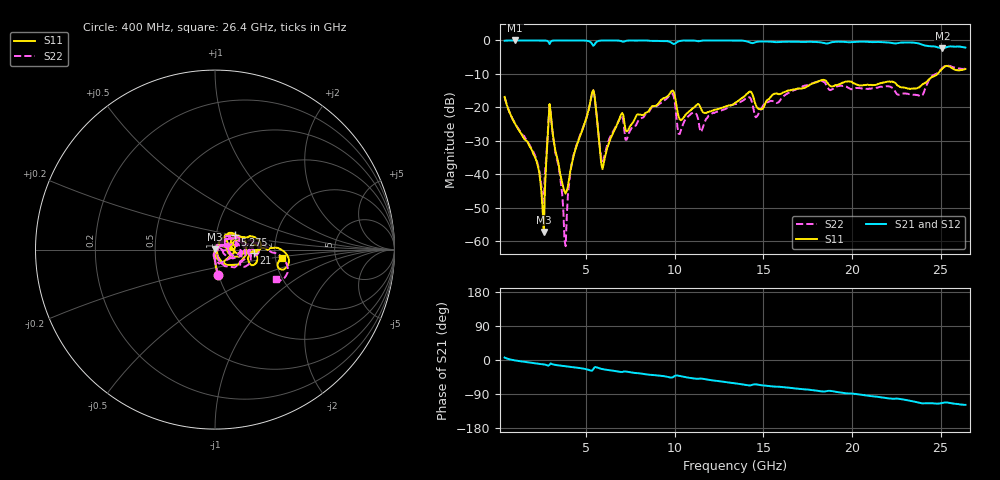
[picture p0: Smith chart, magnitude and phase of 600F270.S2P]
!  American Technical Ceramics  Date:  11/23/05
!  One Norden Lane
!  Huntington Station,  NY.  11746-2102
!  Tel:  (631) 622-4700  Fax:  (631) 622-4748
!  Part Number  600F270  Mounting Orientation: Horizontal
!  Description: Ultra Low ESR Microwave capacitors
!  Application: Coupling, Bypass, Tuning, DC Block
!  Filters, Matching
# GHZ S DB R 50
! Freq  |S11|  S11 Ph  |S21|  S21 Ph  |S12|  S12 Ph  |S22|  S22 Ph
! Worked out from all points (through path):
!   401 points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, 400 MHz to 26.4 GHz, reference 50 ohm
!   highest |S21| = 0.00 dB at 985 MHz (marker M1); lowest = -2.3 dB at 25.1 GHz (marker M2)
!   group delay of S21, straight-line fit = 12.9 ps
!   lowest |S11| = -57.1 dB at 2.61 GHz (marker M3), VSWR 1.00, Z = 50.1 + j0.0747 ohm
!   |S11| at or under -10 dB: start of sweep to 24.83 GHz
!   |S22| runs from -61.4 to -7.5 dB; largest |S21 - S12| = 0.0068
!   S11 on the Smith chart (normalised r, x): 400 MHz: 0.99, -0.29; 5.275 GHz: 1.23, +0.20; 21 GHz: 1.55, -0.06; 26.4 GHz: 2.16, -0.25
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0.4  -16.85 -83.4  -0.08 6.5  -0.08 6.5  -16.85 -83.2
0.985  -24.82 -91.1  0.00 -1.1  -0.01 -1.1  -24.72 -89.9
2.09  -34.56 -99.9  -0.01 -8.3  -0.01 -8.3  -34.05 -94.9
2.61  -57.15 32.5  -0.02 -11.6  -0.02 -11.7  -47.26 15.6
3  -21.52 -60.9  -0.39 -9.1  -0.41 -9.3  -21.74 -73.6
3.845  -45.71 -2.8  -0.01 -16.6  -0.01 -16.7  -61.40 60.2
4.235  -35.88 62.5  -0.01 -18.8  0.00 -18.8  -35.54 71.8
4.755  -27.19 62.3  -0.01 -22.1  -0.03 -22.1  -27.01 56.7
5.275  -17.28 35.8  -0.61 -28.2  -0.62 -28.1  -17.36 26.6
5.99  -36.68 20.9  -0.01 -24.7  -0.01 -24.7  -35.45 5.7
6.965  -22.18 46.6  -0.18 -31.5  -0.18 -31.5  -22.78 22.8
7.355  -26.88 42.7  -0.04 -31.3  -0.04 -31.3  -28.58 36.0
9.11  -18.58 50.6  -0.17 -41.5  -0.17 -41.5  -19.05 42.3
9.825  -15.10 16.8  -0.70 -46.3  -0.69 -46.2  -15.73 9.9
10.28  -23.54 -3.2  -0.18 -42.3  -0.18 -42.4  -27.93 15.9
13.4  -18.66 23.4  -0.01 -61.2  -0.01 -61.4  -18.99 27.6
17.755  -12.87 18.2  -0.43 -79.6  -0.44 -79.8  -12.80 9.9
21.005  -13.32 -4.6  -0.47 -95.0  -0.43 -95.2  -14.33 -4.4
22.11  -12.25 -14.2  -0.67 -101.5  -0.69 -101.6  -13.75 -22.5
23.865  -13.66 -2.9  -1.06 -113.7  -1.07 -113.8  -16.65 -8.1
25.1  -8.40 -1.0  -2.29 -113.4  -2.30 -113.6  -8.22 -7.6
26.4  -8.53 -7.6  -2.12 -118.3  -2.10 -118.5  -8.42 -25.6
